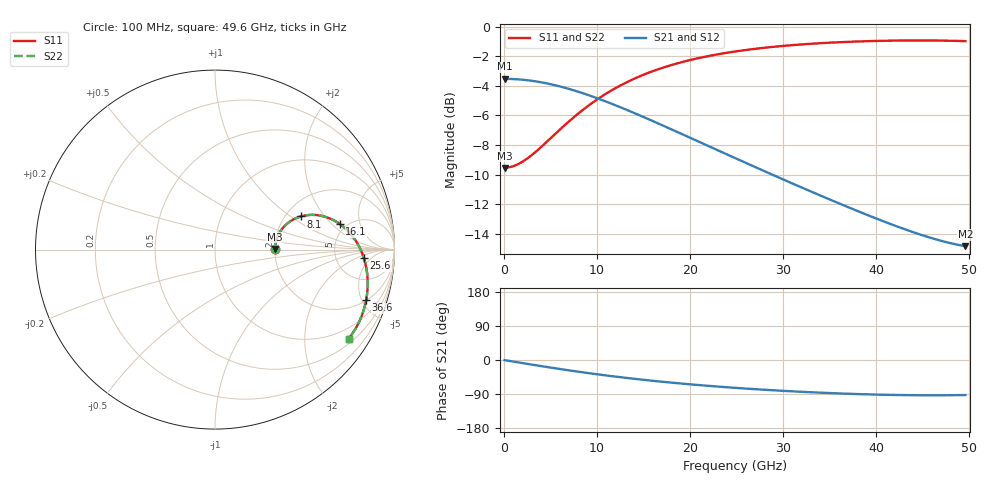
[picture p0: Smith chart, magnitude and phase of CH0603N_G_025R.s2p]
# GHz S RI R 25
! S-Parameters data
! Freq  reS11  imS11  reS21  imS21  reS12  imS12  reS22  imS22
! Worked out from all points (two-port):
!   100 points, 100 MHz to 49.6 GHz, reference 25 ohm
!   highest |S21| = -3.52 dB at 100 MHz (marker M1); lowest = -14.8 dB at 49.6 GHz (marker M2)
!   |S21| within 3 dB of the highest: start of sweep to 16.54 GHz
!   lowest |S11| = -9.5 dB at 100 MHz (marker M3), VSWR 2.00, Z = 50 + j0.353 ohm
!   |S11| at or under -10 dB: nowhere
!   |S22| runs from -9.5 to -0.9 dB; largest |S21 - S12| = 0
!   S11 on the Smith chart (normalised r, x): 100 MHz: 2.00, +0.01; 8.1 GHz: 2.40, +1.20; 16.1 GHz: 4.36, +2.52; 25.6 GHz: 10, -3; 36.6 GHz: 2.02, -5.39; 49.6 GHz: 0.65, -3.19
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0.1  0.3334 0.00314  0.6666 -0.00471  0.6666 -0.00471  0.3334 0.00314
1.6  0.3401 0.0496  0.6595 -0.0747  0.6595 -0.0747  0.3401 0.0496
3.6  0.3666 0.1059  0.6318 -0.1624  0.6318 -0.1624  0.3666 0.1059
6.1  0.4219 0.1593  0.5736 -0.2549  0.5736 -0.2549  0.4219 0.1593
8.1  0.4769 0.1844  0.515 -0.3111  0.515 -0.3111  0.4769 0.1844
8.6  0.4914 0.1882  0.4995 -0.3226  0.4995 -0.3226  0.4914 0.1882
10.1  0.5355 0.1935  0.452 -0.3512  0.452 -0.3512  0.5355 0.1935
12.1  0.5932 0.188  0.3889 -0.3764  0.3889 -0.3764  0.5932 0.188
14.1  0.6467 0.1705  0.329 -0.3893  0.329 -0.3893  0.6467 0.1705
16.1  0.6944 0.1435  0.2742 -0.3924  0.2742 -0.3924  0.6944 0.1435
16.6  0.7052 0.1356  0.2614 -0.392  0.2614 -0.392  0.7052 0.1356
18.6  0.7443 0.1003  0.2139 -0.3864  0.2139 -0.3864  0.7443 0.1003
20.6  0.7766 0.0607  0.1724 -0.376  0.1724 -0.376  0.7766 0.0607
22.6  0.8023 0.0184  0.1366 -0.3625  0.1366 -0.3625  0.8023 0.0184
25.1  0.8259 -0.0365  0.0993 -0.343  0.0993 -0.343  0.8259 -0.0365
25.6  0.8296 -0.0476  0.0927 -0.3389  0.0927 -0.3389  0.8296 -0.0476
29.1  0.8467 -0.1252  0.054 -0.3092  0.054 -0.3092  0.8467 -0.1252
33.1  0.8502 -0.2113  0.0232 -0.2757  0.0232 -0.2757  0.8502 -0.2113
36.6  0.8418 -0.2825  0.00553 -0.2485  0.00553 -0.2485  0.8418 -0.2825
41.6  0.8149 -0.3754  -0.0078 -0.215  -0.0078 -0.215  0.8149 -0.3754
46.1  0.7786 -0.448  -0.0104 -0.1922  -0.0104 -0.1922  0.7786 -0.448
49.6  0.7443 -0.4954  -0.0078 -0.1811  -0.0078 -0.1811  0.7443 -0.4954
